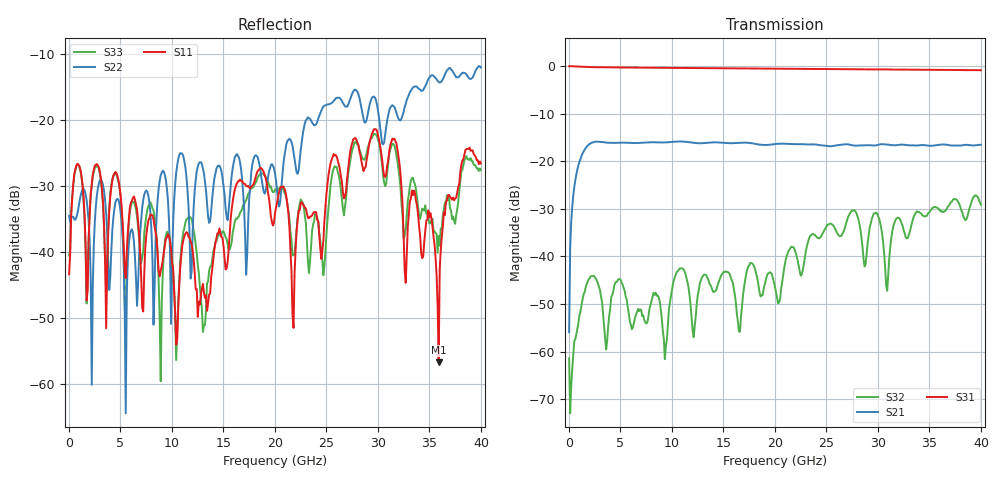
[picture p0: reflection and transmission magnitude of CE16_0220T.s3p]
!Keysight Technologies,N5245A,MY52451697,A.10.60.06
!Date: Thursday, December 02, 2021 17:37:24
!Correction: S11(Full 4 Port(1,2,3,4))
!S13(Full 4 Port(1,2,3,4))
!S14(Full 4 Port(1,2,3,4))
!S31(Full 4 Port(1,2,3,4))
!S33(Full 4 Port(1,2,3,4))
!S34(Full 4 Port(1,2,3,4))
!S41(Full 4 Port(1,2,3,4))
!S43(Full 4 Port(1,2,3,4))
!S44(Full 4 Port(1,2,3,4))
!S3P File: Measurements: <S11,S13,S14>,
!<S31,S33,S34>,
!<S41,S43,S44>:
# Hz S  dB  R 50
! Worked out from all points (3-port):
!   401 points, 10 MHz to 40 GHz, reference 50 ohm
!   strongest paths, dB at 10 MHz, 10.01 GHz, 20 GHz, 30 GHz, 40 GHz:
!     S31: 0.0, -0.4, -0.5, -0.7, -0.9
!     S21: -55.9, -15.9, -16.4, -16.6, -16.5
!     S32: -61.4, -46.9, -46.3, -31.5, -29.1
!   lowest |S11| = -56.8 dB at 35.9 GHz (marker M1), VSWR 1.00, Z = 49.9 + j0.111 ohm
!   |S11| at or under -10 dB: start of sweep to end of sweep
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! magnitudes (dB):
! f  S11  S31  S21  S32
! 10 MHz  -43.4  0.0  -55.9  -61.4
! 509.9 MHz  -28.2  -0.1  -25.5  -57.8
! 2.01 GHz  -34.2  -0.2  -16.4  -44.6
! 9.308 GHz  -39.1  -0.4  -16.0  -61.6
! 13.11 GHz  -46.2  -0.4  -16.2  -43.8
! 20 GHz  -34.2  -0.5  -16.4  -46.3
! 24.7 GHz  -38.3  -0.6  -16.7  -34.9
! 29.7 GHz  -21.4  -0.7  -16.7  -30.9
! 35.9 GHz  -56.8  -0.8  -16.6  -30.1
! 40 GHz  -26.6  -0.9  -16.5  -29.1
